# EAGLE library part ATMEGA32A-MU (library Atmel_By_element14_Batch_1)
8-bit Microcontroller with 32K Bytes In-System Programmable Flash
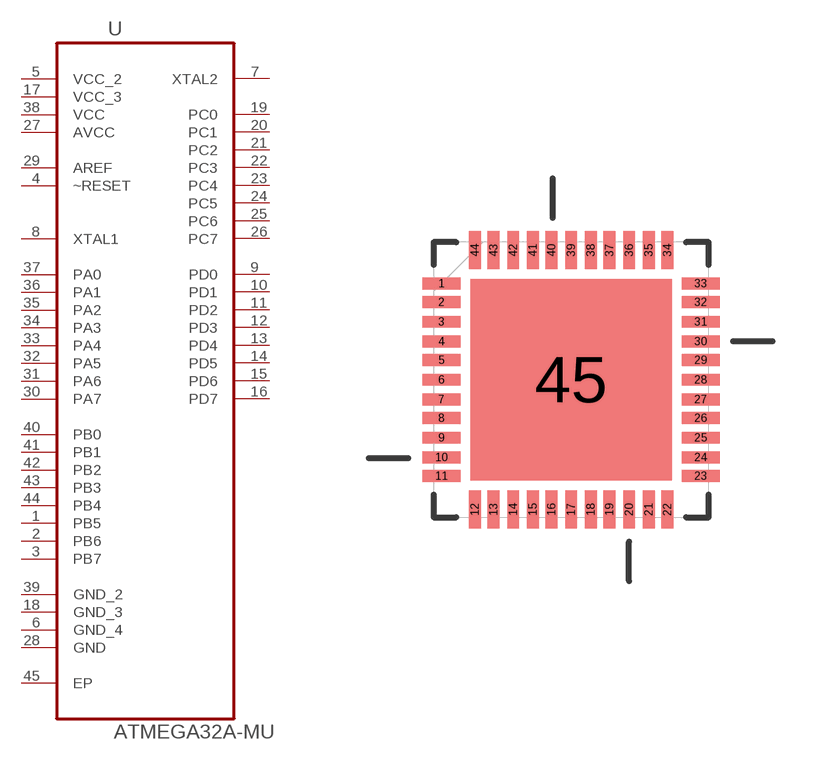
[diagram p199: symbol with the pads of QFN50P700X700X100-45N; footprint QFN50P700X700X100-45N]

Designator prefix U

## ATMEGA32A-MU (MPN: ATMEGA32A-MU; OC_FARNELL: 1748523; OC_NEWARK: 26R5631; PACKAGE: QFN-44; SUPPLIER: Atmel)  [QFN50P700X700X100-45N]
1  PB5
2  PB6
3  PB7
4  ~RESET  in
5  VCC_2  pwr
6  GND_4  pas
7  XTAL2  out
8  XTAL1  in
9  PD0
10  PD1
11  PD2
12  PD3
13  PD4
14  PD5
15  PD6
16  PD7
17  VCC_3  pwr
18  GND_3  pas
19  PC0
20  PC1
21  PC2
22  PC3
23  PC4
24  PC5
25  PC6
26  PC7
27  AVCC  pwr
28  GND  pas
29  AREF  in
30  PA7
31  PA6
32  PA5
33  PA4
34  PA3
35  PA2
36  PA1
37  PA0
38  VCC  pwr
39  GND_2  pas
40  PB0
41  PB1
42  PB2
43  PB3
44  PB4
45  EP  pas

## Footprint QFN50P700X700X100-45N (pad centres in mm)
smd 0.991 x 0.305: 1 -3.353,2.489; 2 -3.353,2.007; 3 -3.353,1.499; 4 -3.353,0.991; 5 -3.353,0.508; 6 -3.353,0; 7 -3.353,-0.508; 8 -3.353,-0.991; 9 -3.353,-1.499; 10 -3.353,-2.007; 11 -3.353,-2.489; 23 3.353,-2.489; 24 3.353,-2.007; 25 3.353,-1.499; 26 3.353,-0.991; 27 3.353,-0.508; 28 3.353,0; 29 3.353,0.508; 30 3.353,0.991; 31 3.353,1.499; 32 3.353,2.007; 33 3.353,2.489
smd 0.305 x 0.991: 12 -2.489,-3.353; 13 -2.007,-3.353; 14 -1.499,-3.353; 15 -0.991,-3.353; 16 -0.508,-3.353; 17 0,-3.353; 18 0.508,-3.353; 19 0.991,-3.353; 20 1.499,-3.353; 21 2.007,-3.353; 22 2.489,-3.353; 34 2.489,3.353; 35 2.007,3.353; 36 1.499,3.353; 37 0.991,3.353; 38 0.508,3.353; 39 0,3.353; 40 -0.508,3.353; 41 -0.991,3.353; 42 -1.499,3.353; 43 -2.007,3.353; 44 -2.489,3.353
smd 5.207 x 5.207: 45 0,0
